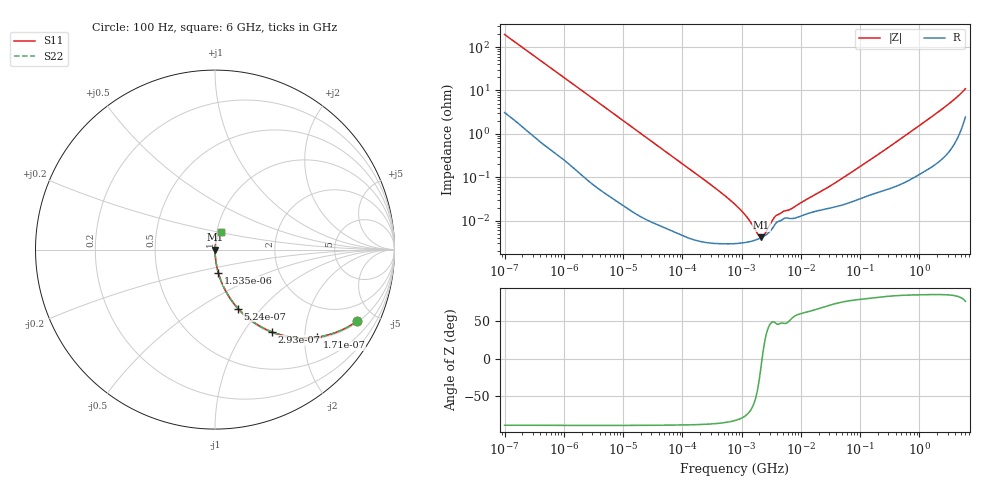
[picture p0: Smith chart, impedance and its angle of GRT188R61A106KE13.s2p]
!Murata Part Number: GRT188R61A106KE13
!These Parameters are Measured in Series Mode Connection
!Data Generated on Jun 19, 2026
!  o--ll--o
!Port1  Port2
!  o------o
!Operation Temp=25[degC], DC Bias Voltage=0[V]
!Freq. Start=100[Hz] Stop=6[GHz] 401[Steps]
# Hz S RI R 50
!Freq.(Hz) S11(Real) S11(Imag) S21(Real) S21(Imag) S12(Real) S12(Imag) S22(Real) S22(Imag)
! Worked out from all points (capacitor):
!   401 points, 100 Hz to 6 GHz, reference 50 ohm
!   read as one part in series: C = 8.1 uF near 109 Hz
!   lowest |Z| = 4.09 mohm at 2.169 MHz (marker M1)
!   series resonance near 2.22 MHz, so ESL is about 630 pH
!   S11 on the Smith chart (normalised r, x): 100 Hz: 1.06, -3.91; 171 Hz: 1.03, -2.30; 293 Hz: 1.02, -1.35; 524 Hz: 1.01, -0.76; 1.535 kHz: 1.00, -0.26; 6 GHz: 1.05, +0.21
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100  0.7892 -0.4  0.2108 0.4  0.2108 0.4  0.7892 -0.4
120  0.7257 -0.4384  0.2743 0.4384  0.2743 0.4384  0.7257 -0.4384
171  0.5685 -0.4878  0.4315 0.4878  0.4315 0.4878  0.5685 -0.4878
293  0.3156 -0.458  0.6844 0.458  0.6844 0.458  0.3156 -0.458
524  0.1288 -0.3286  0.8712 0.3286  0.8712 0.3286  0.1288 -0.3286
820  0.0584 -0.2282  0.9416 0.2282  0.9416 0.2282  0.0584 -0.2282
1535  0.0182 -0.128  0.9818 0.128  0.9818 0.128  0.0182 -0.128
2008  0.011 -0.0988  0.989 0.0988  0.989 0.0988  0.011 -0.0988
6433  0.00132 -0.0314  0.9987 0.0314  0.9987 0.0314  0.00132 -0.0314
40335  0.000103 -0.00506  0.9999 0.00506  0.9999 0.00506  0.000103 -0.00506
316350  3.04e-05 -0.00064  1 0.00064  1 0.00064  3.04e-05 -0.00064
774597  2.95e-05 -0.000235  1 0.000235  1 0.000235  2.95e-05 -0.000235
1386327  3.28e-05 -9.1e-05  1 9.1e-05  1 9.1e-05  3.28e-05 -9.1e-05
2169299  4.07e-05 -4.3e-06  1 4.3e-06  1 4.3e-06  4.07e-05 -4.3e-06
3103719  5.89e-05 6.44e-05  0.9999 -6.44e-05  0.9999 -6.44e-05  5.89e-05 6.44e-05
4856642  0.000105 0.000117  0.9999 -0.000117  0.9999 -0.000117  0.000105 0.000117
6948629  0.000111 0.000151  0.9999 -0.000151  0.9999 -0.000151  0.000111 0.000151
1.555665e7  0.000156 0.000328  0.9998 -0.000328  0.9998 -0.000328  0.000156 0.000328
4.165952e7  0.000214 0.000774  0.9998 -0.000774  0.9998 -0.000774  0.000214 0.000774
3.124326e8  0.000566 0.00501  0.9994 -0.00501  0.9994 -0.00501  0.000566 0.00501
2.240541e9  0.00354 0.0341  0.9965 -0.0341  0.9965 -0.0341  0.00354 0.0341
6e9  0.0345 0.1007  0.9655 -0.1007  0.9655 -0.1007  0.0345 0.1007
